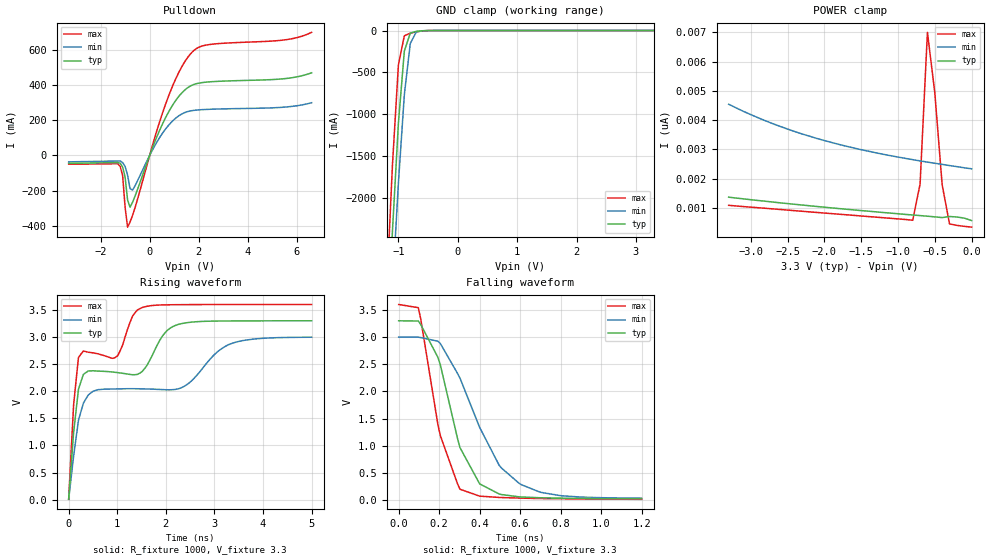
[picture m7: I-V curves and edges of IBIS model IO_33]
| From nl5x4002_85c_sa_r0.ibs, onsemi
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[Model]   IO_33
Model_type I/O_open_drain
Enable Active-High
Polarity Non-Inverting
Vinh=2.31
Vinl=0.99
Vref=3.3
Vmeas=1.65
Rref=1000
Cref=50p
C_comp   6.0p   NA   NA
[Model Spec]
Vinh   2.31   2.10   2.52
Vinl   0.99   0.90   1.08
Vmeas   1.65   1.50   1.80
[Temperature Range] 25   85   -40
[Voltage Range]   3.3   3.0   3.6
[POWER Clamp Reference]  3.3   3.0   3.6
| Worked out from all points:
|   slope of the pulldown table from 0 to 0.495 V, typ, clamps not added: 2.9 ohm
|   GND clamp passes 1 mA (typ) near -0.51 V on its own axis
|   falling waveform, R_fixture 1000, V_fixture 3.3: 20-80 % time 153ps typ, 220ps min, 121ps max; typ from 3.3 V to 0.021 V
|   rising waveform, R_fixture 1000, V_fixture 3.3: 20-80 % time 1.65ns typ, 2.66ns min, 1.08ns max; typ from 0.009 V to 3.3 V
[Pulldown]
-3.3V     -44.48mA   -36.44mA   -49.64mA
-1.3V     -40.53mA   -31.73mA   -46.91mA
-1.1V     -66.63mA   -40.61mA   -116mA
-1V       -123.4mA   -62.34mA   -294.9mA
-900mV    -253mA     -112mA     -408.1mA
-800mV    -294.4mA   -188.2mA   -379.7mA
-700mV    -267.3mA   -197.5mA   -342.2mA
700mV     228.8mA    159.6mA    311.5mA
1.2V      338.3mA    226.7mA    476mA
1.7V      398.2mA    254.5mA    583.7mA
2.3V      417.3mA    261.9mA    628.3mA
6.6V      470.5mA    300mA      700.8mA
[GND Clamp]
-3.3V     -35.42A    -33.28A    -38.2A
-1.2V     -3.822A    -4.412A    -3.136A
-1.1V     -2.385A    -3.071A    -1.6A
-1V       -1.105A    -1.818A    -410.1mA
-900mV    -244.1mA   -763.4mA   -62.39mA
-800mV    -31.41mA   -154.3mA   -31.83mA
-700mV    -10.05mA   -17.99mA   -15.56mA
-600mV    -3.32mA    -2.981mA   -4.628mA
-400mV    -64.31uA   -78.67uA   -39.34uA
3.3V      569.3pA    2.336nA    347.9pA
[POWER Clamp]
-3.3V     1.369nA    4.542nA    1.091nA
-2.7V     1.202nA    3.877nA    968.1pA
-2.1V     1.05nA     3.373nA    846.4pA
-1.5V     910.7pA    2.99nA     726.3pA
-800mV    760.9pA    2.65nA     580.3pA
-700mV    739.7pA    2.607nA    1.813nA
-600mV    718.5pA    2.566nA    6.998nA
-500mV    696.3pA    2.526nA    4.939nA
-400mV    671.9pA    2.489nA    1.793nA
-300mV    708.2pA    2.448nA    456.6pA
-100mV    653.7pA    2.372nA    373.1pA
0V        570pA      2.337nA    344.8pA
[Falling Waveform]
R_fixture=1000
V_fixture=3.3
V_fixture_min=3.0
V_fixture_max=3.6
0s        3.3V       3V         3.6V
96.97ps   3.296V     2.998V     3.542V
193.9ps   2.625V     2.924V     1.384V
206.1ps   2.485V     2.879V     1.181V
303ps     962.8mV    2.242V     196.8mV
400ps     296.4mV    1.336V     70.29mV
497ps     108.9mV    634.8mV    46.14mV
593.9ps   58.32mV    310mV      34.41mV
800ps     33.21mV    78.76mV    22.27mV
1.2ns     20.93mV    31.92mV    11.45mV
[Rising Waveform]
R_fixture=1000
V_fixture=3.3
V_fixture_min=3.0
V_fixture_max=3.6
0s        8.532mV    10.65mV    7.089mV
101ps     1.232V     798.9mV    1.741V
202ps     2.037V     1.465V     2.623V
303ps     2.31V      1.78V      2.742V
959.6ps   2.349V     2.043V     2.624V
1.313ns   2.305V     2.047V     3.382V
1.616ns   2.485V     2.042V     3.568V
2.273ns   3.237V     2.05V      3.597V
3.333ns   3.297V     2.875V     3.6V
5ns       3.3V       2.996V     3.6V
[Ramp]
R_load=1000
dV/dt_r   1.975E+0/1.404E-10   1.793E+0/2.051E-10   2.156E+0/1.498E-10
dV/dt_f   1.967E+0/1.534E-10   1.781E+0/2.192E-10   2.153E+0/1.207E-10
|[End   IO_33
